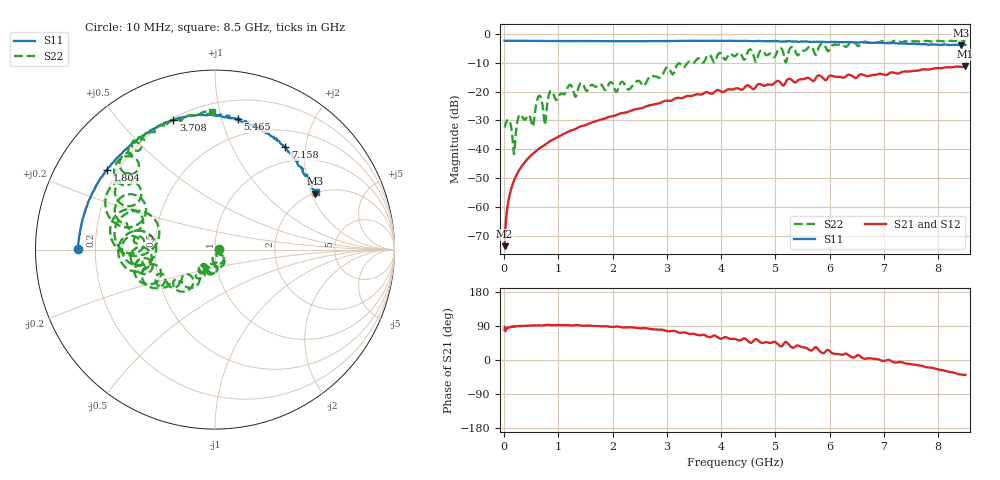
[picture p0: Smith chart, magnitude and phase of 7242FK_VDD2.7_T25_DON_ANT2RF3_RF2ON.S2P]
!Agilent Technologies,E5071C,MY46417908,A.11.23
!Date: Wed Dec 09 15:39:18 2020
!Data & Calibration Information:
!Freq	S11:SOLT2(ON)	S21:SOLT2(ON)	S12:SOLT2(ON)	S22:SOLT2(ON)
!PortZ  Port1:50+j0  Port2:50+j0
!Above PortZ is port z conversion or system Z0 setting when saving the data.
!When reading, reference impedance value at option line is always used.
# Hz S dB R 50
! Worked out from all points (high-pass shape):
!   1601 points, 10 MHz to 8.5 GHz, reference 50 ohm
!   highest |S21| = -11.26 dB at 8.5 GHz (marker M1); lowest = -73.6 dB at 10 MHz (marker M2)
!   |S21| within 3 dB of the highest: 6.806 GHz to 7.029 GHz (223.3 MHz wide, 3.23 % of centre); 7.043 GHz to end of sweep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
!   lowest |S11| = -3.9 dB at 8.42 GHz (marker M3), VSWR 4.52, Z = 101 + j106 ohm
!   |S11| at or under -10 dB: nowhere
!   |S22| runs from -41.6 to -2.3 dB; largest |S21 - S12| = 0.0032
!   S11 on the Smith chart (normalised r, x): 10 MHz: 0.13, +0.00; 1.804 GHz: 0.16, +0.32; 3.708 GHz: 0.21, +0.71; 5.465 GHz: 0.35, +1.13; 7.158 GHz: 0.74, +1.64; 8.5 GHz: 1.99, +2.19
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1e7  -2.32 179.7  -73.59 79.5  -74.74 77.4  -32.47 3.1
8.42875e7  -2.36 178.1  -57.57 86.1  -57.39 85.5  -29.73 -33.6
1.851062e8  -2.38 176.0  -50.72 88.3  -50.84 88.2  -41.64 -30.1
3.230688e8  -2.40 173.1  -45.94 89.8  -45.96 89.6  -28.24 -54.0
5.247062e8  -2.40 169.1  -41.65 90.7  -41.65 91.0  -32.05 -59.6
6.520562e8  -2.42 166.7  -39.65 91.4  -39.65 91.5  -21.44 -72.4
7.52875e8  -2.44 164.6  -38.48 92.0  -38.49 92.1  -31.60 -72.1
8.59e8  -2.44 162.3  -37.04 92.1  -37.04 92.1  -19.78 -71.1
1.320644e9  -2.48 153.1  -32.93 91.9  -32.94 92.0  -21.75 -98.2
1.426769e9  -2.47 151.3  -31.96 90.6  -31.96 90.6  -16.96 -105.1
1.803512e9  -2.53 143.7  -29.60 88.8  -29.60 88.8  -17.82 -122.6
2.843538e9  -2.48 122.1  -24.10 80.3  -24.11 80.3  -15.10 -126.0
3.708456e9  -2.42 107.8  -20.28 65.0  -20.28 65.0  -8.87 -145.7
4.255e9  -2.46 99.1  -18.99 55.6  -18.99 55.6  -7.72 -169.3
5.464825e9  -2.63 80.0  -15.72 35.0  -15.69 35.1  -6.30 166.8
5.671769e9  -2.75 76.7  -16.11 25.7  -16.05 25.6  -4.62 149.1
5.777894e9  -2.68 76.5  -14.49 29.6  -14.50 29.8  -5.70 166.1
5.899938e9  -2.81 73.9  -15.78 19.1  -15.72 19.2  -3.78 143.1
7.088538e9  -3.18 56.6  -13.75 0.4  -13.81 0.3  -3.15 127.0
7.157519e9  -3.17 55.6  -13.32 -4.7  -13.33 -4.6  -2.58 128.6
8.420406e9  -3.91 29.3  -11.46 -38.4  -11.52 -38.6  -2.28 93.6
8.5e9  -3.76 29.4  -11.26 -39.6  -11.34 -39.5  -2.32 91.1
